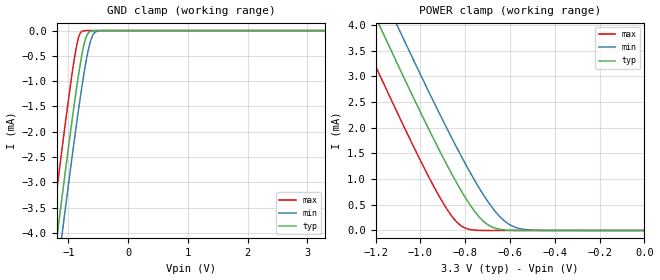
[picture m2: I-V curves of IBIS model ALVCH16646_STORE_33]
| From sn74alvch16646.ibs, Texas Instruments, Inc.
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[Model]   ALVCH16646_STORE_33
Model_type  Input
Vinl=0.8
Vinh=2.0
| variable   typ   min   max
C_comp   1.61pF   1.38pF   2.22pF
[Temperature Range]   40   100   -40
| Ambient temperature   25   85   -40
[Voltage range]   3.3   3   3.6
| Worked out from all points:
|   GND clamp passes 1 mA (typ) near -0.85 V on its own axis
|   POWER clamp passes 1 mA (typ) near -0.85 V on its own axis
[GND Clamp]
| ALVCH16646_STORE_33
|   Voltage   I(typ)   I(min)   I(max)
-3.3V     -24.83mA   -25.52mA   -23.96mA
-1.3V     -5.111mA   -5.849mA   -4.158mA
-1.26V    -4.729mA   -5.468mA   -3.775mA
-1.185V   -4.018mA   -4.758mA   -3.062mA
-1.09V    -3.13mA    -3.869mA   -2.175mA
-880mV    -1.265mA   -1.975mA   -406.2uA
-825mV    -828.8uA   -1.509mA   -114.4uA
-770mV    -446.6uA   -1.069mA   -12.88uA
-700mV    -116.1uA   -571.7uA   -455.3nA
-630mV    -13.33uA   -205.5uA   -15.19nA
-500mV    -126.5nA   -7.204uA   -35.76pA
3.3V      6.303pA    16.94nA    5.63pA
[POWER Clamp]
| ALVCH16646_STORE_33
|   Voltage   I(typ)   I(min)   I(max)
-3.3V     24.83mA    25.52mA    23.96mA
-1.275V   4.872mA    5.61mA     3.918mA
-1.185V   4.018mA    4.758mA    3.062mA
-1.105V   3.269mA    4.008mA    2.314mA
-1.07V    2.945mA    3.683mA    1.992mA
-940mV    1.776mA    2.501mA    856.4uA
-845mV    982.9uA    1.676mA    200.1uA
-795mV    611.2uA    1.266mA    38.41uA
-725mV    207uA      738.7uA    1.527uA
-625mV    11.21uA    186.8uA    11.91nA
-510mV    181.6nA    9.688uA    52.91pA
-48.03fV  6.303pA    7.801pA    6.677pA
